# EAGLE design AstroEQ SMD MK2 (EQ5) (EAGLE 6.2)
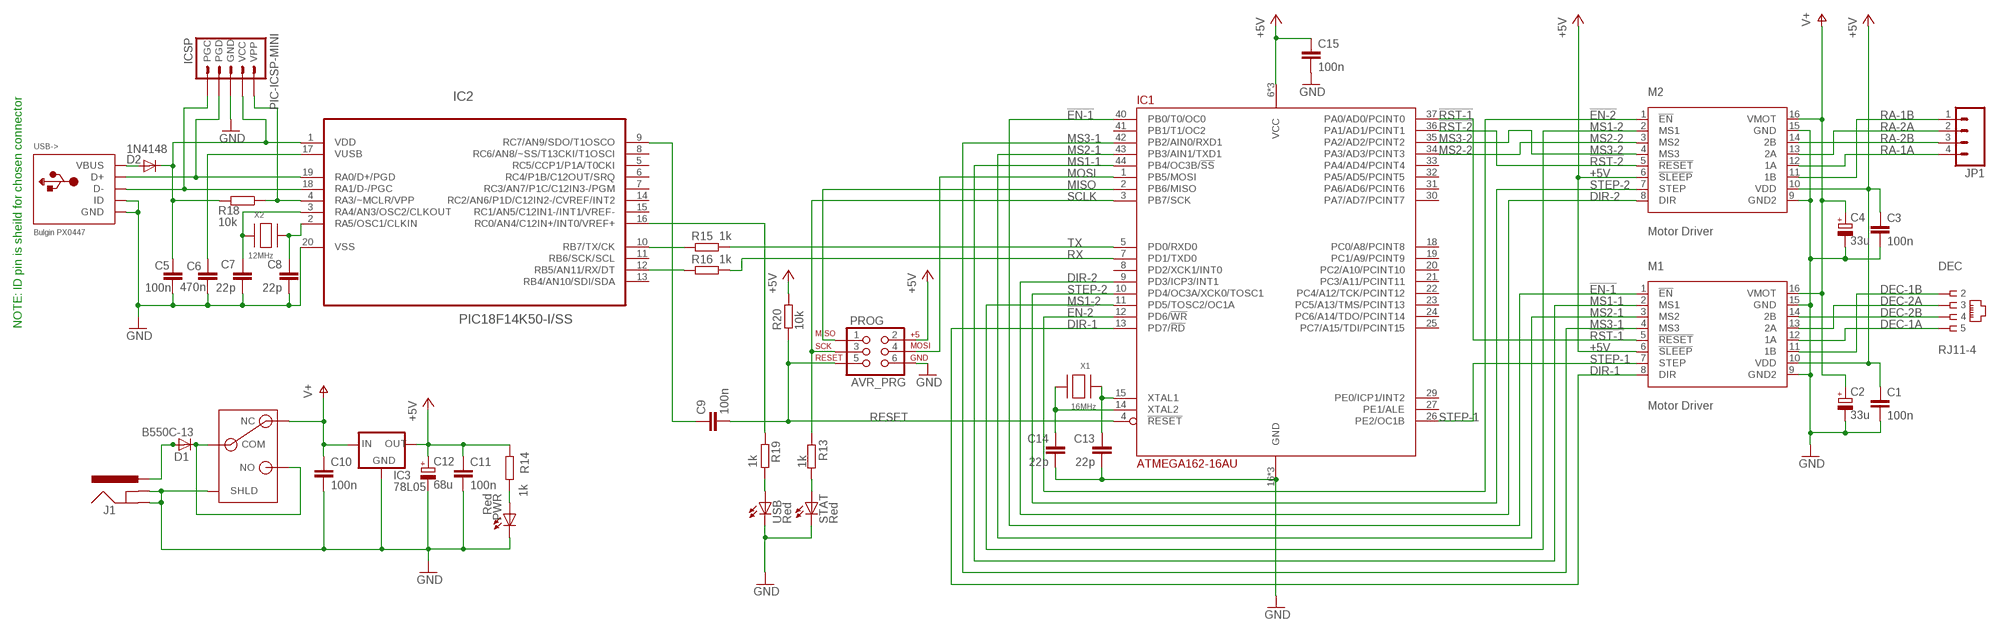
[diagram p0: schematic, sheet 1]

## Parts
C1  100n  C-EUC0603  [C0603]
C2  33u  CPOL-EUC/6032-28R  [C/6032-28R]
C3  100n  C-EUC0603  [C0603]
C4  33u  CPOL-EUC/6032-28R  [C/6032-28R]
C5  100n  C-EUC0603  [C0603]
C6  470n  C-EUC0603  [C0603]
C7  22p  C-EUC0603  [C0603]
C8  22p  C-EUC0603  [C0603]
C9  100n  C-EUC0603  [C0603]
C10  100n  C-EUC0603  [C0603]
C11  100n  C-EUC0603  [C0603]
C12  68u  CPOL-EUC/6032-28R  [C/6032-28R]
C13  22p  C-EUC0603  [C0603]
C14  22p  C-EUC0603  [C0603]
C15  100n  C-EUC0603  [C0603]
D1  B550C-13  DIODE-SMC  [SMC]
D2  1N4148  DIODESOD  [SOD-323]
DEC  RJ11-4  [RJ11-NO_SHIELD-4]
IC1  ATMEGA162-16AU  [TQFP44]
IC2  PIC18F14K50-I/SS  [SS20]
IC3  78L05  78LXXSOT-23  [SOT23]
ICSP  PIC-ICSP-MINI  [PIC-ICSP-MINI]
J1  POWER_JACKPANEL  [POWER_JACK_PANEL]
JP1  M04POLAR  [MOLEX-1X4]
M1  Motor Driver  A4983CARRIER  [DIP16-W]
M2  Motor Driver  A4983CARRIER  [DIP16-W]
PROG  AVR_PRG  AVR_SPI_PRG_6PTH  [2X3]
PWR  Red  LED3MM  [LED3MM]
R13  1k  R-EU_R0603  [R0603]
R14  1k  R-EU_R0603  [R0603]
R15  1k  R-EU_R0603  [R0603]
R16  1k  R-EU_R0603  [R0603]
R18  10k  R-EU_R0603  [R0603]
R19  1k  R-EU_R0603  [R0603]
R20  10k  R-EU_R0603  [R0603]
STAT  Red  LED3MM  [LED3MM]
SW1  SWITCH  [SPST]
USB  Red  LED3MM  [LED3MM]
USB->  Bulgin PX0447  USBBULGIN  [USB-MINIB-BULGIN]
X1  16MHz  XTALNX5032  [NX5032]
X2  12MHz  XTALNX5032  [NX5032]

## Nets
!EN-1: IC1.40(PB0/T0/OC0) M1.1(!EN)
!EN-2: IC1.12(PD6/!WR) M2.1(!EN)
!RST-1: IC1.37(PA0/AD0/PCINT0) M1.5(!RESET)
!RST-2: IC1.36(PA1/AD1/PCINT1) M2.5(!RESET)
+5V: C1.1 C3.1 C11.1 C12.+ C15.1 IC1.6(VCC) IC1.17(VCC) IC1.38(VCC) IC3.1(OUT) M1.6(!SLEEP) M1.10(VDD) M2.6(!SLEEP) M2.10(VDD) PROG.2 R14.1 R20.2
AVROSC1: C13.1 IC1.15(XTAL1) X1.P$1
AVROSC2: C14.1 IC1.14(XTAL2) X1.P$2
D+: IC2.19(RA0/D+/PGD) ICSP.4(PGD) USB->.3(D+)
D-: IC2.18(RA1/D-/PGC) ICSP.5(PGC) USB->.2(D-)
DEC-1A: DEC.5 M1.12(1A)
DEC-1B: DEC.2 M1.11(1B)
DEC-2A: DEC.3 M1.13(2A)
DEC-2B: DEC.4 M1.14(2B)
DIR-1: IC1.13(PD7/!RD) M1.8(DIR)
DIR-2: IC1.9(PD3/ICP3/INT1) M2.8(DIR)
DTR: C9.1 IC2.9(RC7/AN9/SDO/T1OSCO)
GND: C1.2 C2.- C3.2 C4.- C5.2 C6.1 C7.2 C8.2 C10.2 C11.2 C12.- C13.2 C14.2 C15.2 IC1.16(GND) IC1.28(GND) IC1.39(GND) IC2.20(VSS) IC3.3(GND) ICSP.3(GND) J1.SHUNT(GNDBREAK) J1.SLEEVE(GND) M1.9(GND2) M1.15(GND) M2.9(GND2) M2.15(GND) PROG.6 PWR.K(C) STAT.K(C) SW1.S1(SHLD) SW1.S2(SHLD) SW1.S3(SHLD) SW1.S4(SHLD) USB->.4(GND) USB->.5(ID) USB.K(C)
MCLR: IC2.4(RA3/~MCLR/VPP) ICSP.1(VPP) R18.1
MISO: IC1.2(PB6/MISO) PROG.1
MOSI: IC1.1(PB5/MOSI) PROG.4
MS1-1: IC1.44(PB4/OC3B/!SS) M1.2(MS1)
MS1-2: IC1.11(PD5/TOSC2/OC1A) M2.2(MS1)
MS2-1: IC1.43(PB3/AIN1/TXD1) M1.3(MS2)
MS2-2: IC1.34(PA3/AD3/PCINT3) M2.3(MS2)
MS3-1: IC1.42(PB2/AIN0/RXD1) M1.4(MS3)
MS3-2: IC1.35(PA2/AD2/PCINT2) M2.4(MS3)
PWRLED: PWR.A R14.2
RA-1A: JP1.4 M2.12(1A)
RA-1B: JP1.1 M2.11(1B)
RA-2A: JP1.2 M2.13(2A)
RA-2B: JP1.3 M2.14(2B)
RESET: C9.2 IC1.4(!RESET) PROG.5 R20.1
RX: IC1.7(PD1/TXD0) R16.1
RX(USB): IC2.12(RB5/AN11/RX/DT) R16.2
SCLK: IC1.3(PB7/SCK) PROG.3 R13.1
STATLED: R13.2 STAT.A
STEP-1: IC1.26(PE2/OC1B) M1.7(STEP)
STEP-2: IC1.10(PD4/OC3A/XCK0/TOSC1) M2.7(STEP)
SWITCH: D1.C SW1.COM SW1.NO
TX: IC1.5(PD0/RXD0) R15.1
TX(USB): IC2.10(RB7/TX/CK) R15.2
USBLED: R19.1 USB.A
USBOSC1: C8.1 IC2.2(RA5/OSC1/CLKIN) X2.P$2
USBOSC2: C7.1 IC2.3(RA4/AN3/OSC2/CLKOUT) X2.P$1
USBSTAT: IC2.16(RC0/AN4/C12IN+/INT0/VREF+) R19.2
V+: C2.+ C4.+ C10.1 IC3.2(IN) M1.16(VMOT) M2.16(VMOT) SW1.NC
VBUS: D2.2(A) USB->.1(VBUS)
VIN: D1.A J1.CENTRE(PWR)
VPIC: C5.1 D2.1(C) IC2.1(VDD) ICSP.2(VCC) R18.2
VUSB: C6.2 IC2.17(VUSB)
Unconnected: IC1.8(PD2/XCK1/INT0) IC1.18(PC0/A8/PCINT8) IC1.19(PC1/A9/PCINT9) IC1.20(PC2/A10/PCINT10) IC1.21(PC3/A11/PCINT11) IC1.22(PC4/A12/TCK/PCINT12) IC1.23(PC5/A13/TMS/PCINT13) IC1.24(PC6/A14/TDO/PCINT14) IC1.25(PC7/A15/TDI/PCINT15) IC1.27(PE1/ALE) IC1.29(PE0/ICP1/INT2) IC1.30(PA7/AD7/PCINT7) IC1.31(PA6/AD6/PCINT6) IC1.32(PA5/AD5/PCINT5) IC1.33(PA4/AD4/PCINT4) IC1.41(PB1/T1/OC2) IC2.5(RC5/CCP1/P1A/T0CKI) IC2.6(RC4/P1B/C12OUT/SRQ) IC2.7(RC3/AN7/P1C/C12IN3-/PGM) IC2.8(RC6/AN8/~SS/T13CKI/T1OSCI) IC2.11(RB6/SCK/SCL) IC2.13(RB4/AN10/SDI/SDA) IC2.14(RC2/AN6/P1D/C12IN2-/CVREF/INT2) IC2.15(RC1/AN5/C12IN1-/INT1/VREF-)

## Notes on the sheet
- NOTE: ID pin is sheild for chosen connector

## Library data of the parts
C1 C3 C5 C9-C11 C15 = resistor:C-EU: CAPACITOR, European symbol; MF: MULTICOMP; MPN: T0603F104ZCT; OC_FARNELL: 9406204
C2 C4 = resistor:CPOL-EU: POLARIZED CAPACITOR, European symbol; MF: KEMET; MPN: T491C336K025AT; OC_FARNELL: 1793896
C6 = rcl:C-EU: CAPACITOR, European symbol; MF: MURATA; MPN: GRM188R61C474KA93D; OC_FARNELL: 1828894
C7 C8 C13 C14 = rcl:C-EU: CAPACITOR, European symbol; MF: MULTICOMP; MPN: U0603C220JCT; OC_FARNELL: 9406107
C12 = resistor:CPOL-EU: POLARIZED CAPACITOR, European symbol; MF: AVX; MPN: TPSC686K016R0125; OC_FARNELL: 1658976
D1 = diode:DIODE-: DIODE; MF: DIODES INC.; MPN: B550C-13-F; OC_FARNELL: 1858608
D2 = SparkFun:DIODE: Diode; MF: VISHAY SEMICONDUCTOR; MPN: 1N4148WS-V-GS08; OC_FARNELL: 1617737
DEC = con-tycoelectronics:RJ11-4; MF: MOLEX; MPN: 95503-2641; OC_FARNELL: 1572017
IC1 = atmel:ATMEGA162: 8-bit RISC MICROCONTROLLER 16K Bytes internal flash program memory 1K Bytes internal SRAM Upto 64K Bytes optional external memory space 512 Bytes EEPROM Two 8-bit timers Two 16-bit timers Dual programmable serial USARTs Master/Slave serial SPI interface Source: ATMEGA162_DIP40.lbr; MF: ATMEL; MPN: ATMEGA162-16AU; OC_FARNELL: 9171150
IC2 = microchip:PIC18F14K50: USB Flash Microcontrollers; MF: MICROCHIP; MPN: PIC18F14K50-I/SS; OC_FARNELL: 1648504; PACKAGE: SSOP20; SUPPLIER: Microchip
IC3 = v-reg:78LXX: VOLTAGE REGULATOR; MF: TAIWAN SEMICONDUCTOR; MPN: TS78L05CX RF; OC_FARNELL: 1476698
ICSP = SparkFun:PIC-ICSP-MINI: PIC-ICSP-Mini Miniature 5-pin connection for temporary programming of PICs. Use this device in your design to save space. Program the PIC with this adapter Spark Fun Electronics SKU : BOB-00194; MF: HARWIN; MPN: M52-5000545; OC_FARNELL: 1099543
J1 = SparkFun:POWER_JACK: Power Jack This is the standard 5.5mm barrel jack for power. The PTH is the most common, proven, reliable, footprint. All others are experimental. The Slot footprint only works if the mill layer is transmitted to the PCB fab house so be warned. Spark Fun Electronics SKU : PRT-00119. Mating wall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; MF: SWITCHCRAFT; MPN: PCL712AS; OC_FARNELL: 1871167
JP1 = SparkFun:M04: Header 4 Standard 4-pin 0.1" header. Use with straight break away headers (SKU : PRT-00116), right angle break away headers (PRT-00553), swiss pins (PRT-00743), machine pins (PRT-00117), and female headers (PRT-00115). Molex polarized connector foot print use with SKU : PRT-08231 with associated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; MF: MULTICOMP; MPN: MC34645; OC_FARNELL: 1675775
M1 M2 = A4983Carrier:A4983CARRIER; OC_FARNELL: unknown
PROG = SparkFun:AVR_SPI_PRG_6: AVR ISP 6 Pin This is the reduced ISP connector for AVR programming. Common on Arduino. This footprint will take up less PCB space and can be used with a 10-pin to 6-pin adapter such as SKU: BOB-08508; MF: TE CONNECTIVITY / AMP; MPN: 826632-3; OC_FARNELL: 3418492
PWR STAT USB = led:LED: LED; MF: KINGBRIGHT; MPN: L-424HDT; OC_FARNELL: 1142499
R13 R14 R19 = rcl:R-EU_: RESISTOR, European symbol; MF: PANASONIC; MPN: ERJ3GEYJ102V; OC_FARNELL: 2059601
R15 R16 = SmartPrj:R-EU_: RESISTOR, European symbol; MF: PANASONIC; MPN: ERJ3GEYJ102V; OC_FARNELL: 2059601
R18 R20 = rcl:R-EU_: RESISTOR, European symbol; MF: PANASONIC; MPN: ERJ3GEYJ103V; OC_FARNELL: 2059627
SW1 = con-tycoelectronics:SWITCH; MF: TE CONNECTIVITY; MPN: AE101J1V3B004; OC_FARNELL: 1813654
USB-> = adafruit:USB: USB Connectors USBMINIB - Surface Mount Female Mini-B USB Connector 4UConnector: 06564 By microbuilder.eu Thru-hole RA Female Mini-B USB Connector 4UConnector: 18732 By ladyada.net; MF: BULGIN; MPN: PX0447; OC_FARNELL: 1229687
X1 = adafruit:XTAL: Low cost SMT crystals, no capacitors included; MF: TXC; MPN: 7A-16.000MAAJ-T; OC_FARNELL: 1841946
X2 = adafruit:XTAL: Low cost SMT crystals, no capacitors included; MF: TXC; MPN: 7A-12.000MAAJ-T; OC_FARNELL: 1841940

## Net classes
1 power: width 0.61 mm, drill 0.711 mm, clearance 0.203 mm
2 gnd: width 0.305 mm, drill 0.711 mm, clearance 0.203 mm
3 usbvcc: width 0.508 mm, drill 0.711 mm, clearance 0.203 mm

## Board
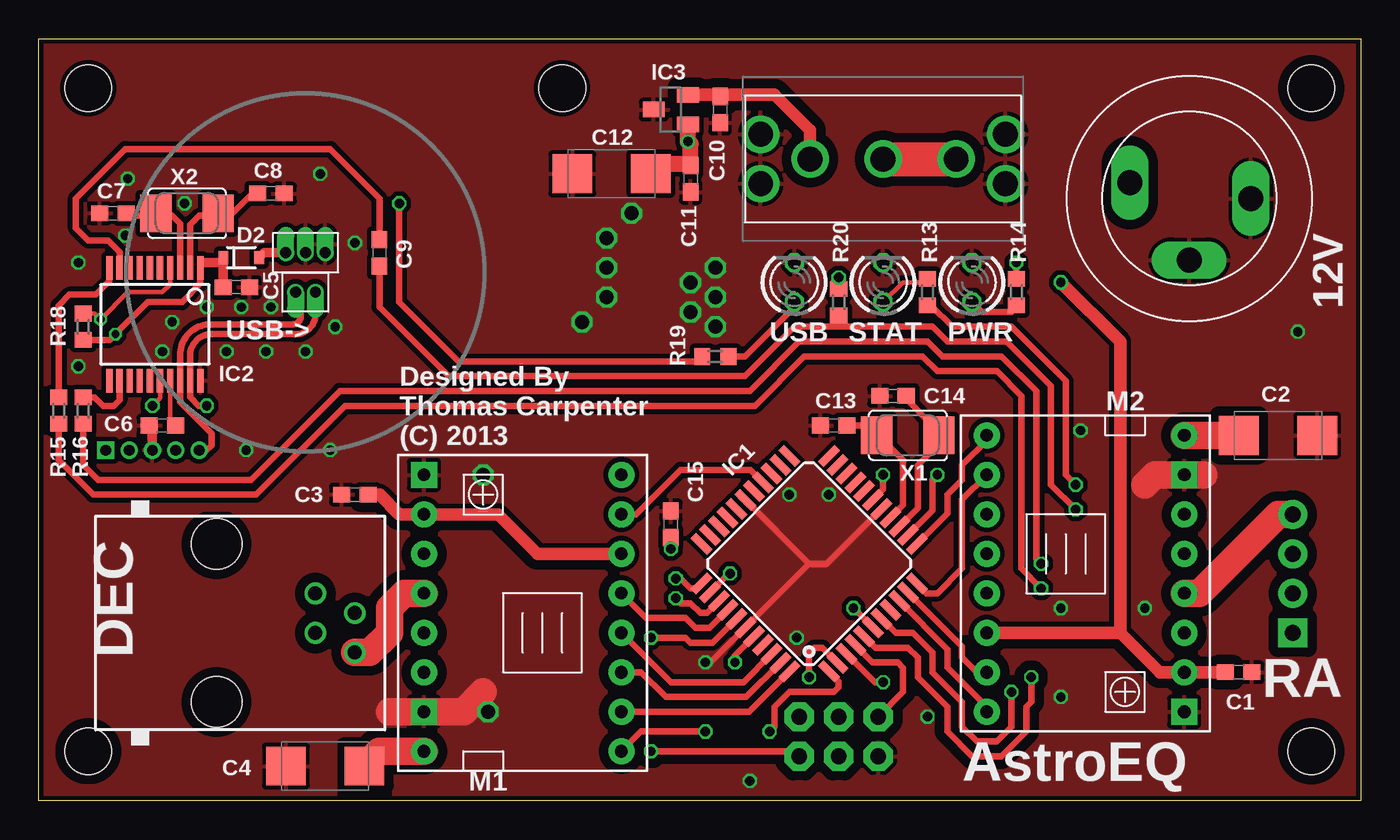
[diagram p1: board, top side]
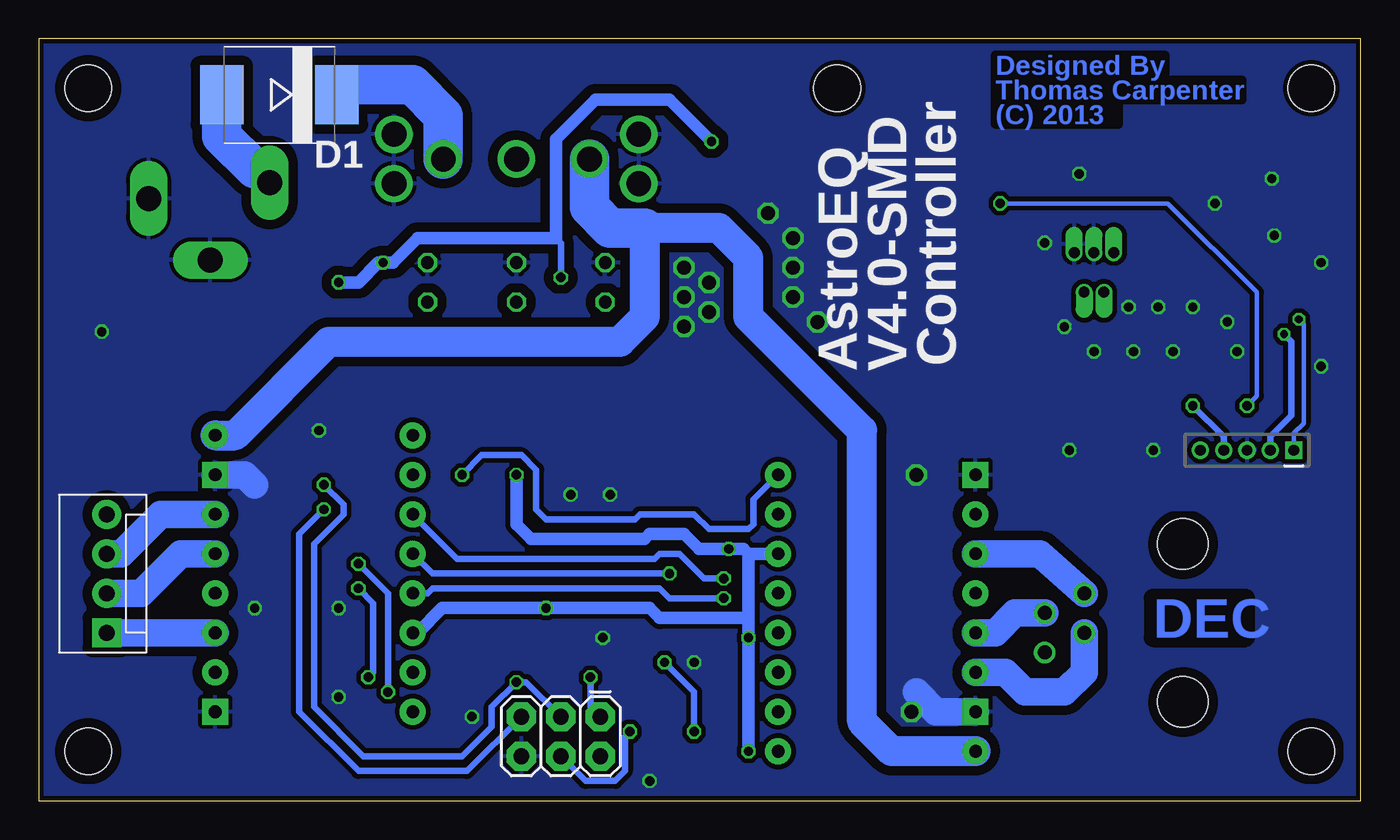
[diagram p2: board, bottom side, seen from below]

Size 85 x 49 mm. Coordinates in mm from the lower left corner, seen from the top.
Outline: 0,0 0,49 85,49 85,0 0,0
Copper layers (1*16): Top 0.035mm / dielectric 1.5mm / Bottom 0.035mm
Design rules: minimum track width 6mil, minimum drill 12mil, track to track 6mil, track to pad 6mil, pad to pad 6mil, via to via 6mil, smd to smd 0mil, copper to edge 10mil, drill to drill 10mil, minimum pad ring 8mil, minimum via ring 6mil, stop-mask expansion 2mil, vias tented up to drill 1mm, thermal gap 10mil
Holes 3 mm at 81.83,3.17 33.66,45.83 3.17,45.83 81.83,45.83 3.17,3.17
tKeepout: area 78.3,7.4 to 83.3,12.4; area 78.3,53.6 to 83.3,58.6; area 48.3,7.4 to 53.3,12.4; area 8.3,7.4 to 13.3,12.4; area 48.3,53.6 to 53.3,58.6; area 8.3,53.6 to 13.3,58.6
bKeepout: area 78.3,7.4 to 83.3,12.4; area 78.3,53.6 to 83.3,58.6; area 48.3,7.4 to 53.3,12.4; area 8.3,7.4 to 13.3,12.4; area 48.3,53.6 to 53.3,58.6; area 8.3,53.6 to 13.3,58.6

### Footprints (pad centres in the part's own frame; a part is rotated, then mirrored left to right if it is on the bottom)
C0603 = smd 1.1 x 1: 1 -0.85,0; 2 0.85,0
C/6032-28R = smd 2.55 x 2.5: + 2.525,0; - -2.525,0
SMC = smd 2.8 x 3.8: A 3.7,0; C -3.7,0
SOD-323 = smd 0.63 x 0.83: 1 -1.15,0; 2 1.15,0
RJ11-NO_SHIELD-4 = drill 0.9 pad 1.4: 2 -1.905,6.35; 3 -0.635,8.89; 4 0.635,6.35; 5 1.905,8.89 | hole 3.251: -5.08,0; 5.08,0
TQFP44 = smd 1.5 x 0.5: 1 -5.8,4; 2 -5.8,3.2; 3 -5.8,2.4; 4 -5.8,1.6; 5 -5.8,0.8; 6 -5.8,0; 7 -5.8,-0.8; 8 -5.8,-1.6; 9 -5.8,-2.4; 10 -5.8,-3.2; 11 -5.8,-4; 23 5.8,-4; 24 5.8,-3.2; 25 5.8,-2.4; 26 5.8,-1.6; 27 5.8,-0.8; 28 5.8,0; 29 5.8,0.8; 30 5.8,1.6; 31 5.8,2.4; 32 5.8,3.2; 33 5.8,4 | smd 0.5 x 1.5: 12 -4,-5.8; 13 -3.2,-5.8; 14 -2.4,-5.8; 15 -1.6,-5.8; 16 -0.8,-5.8; 17 0,-5.8; 18 0.8,-5.8; 19 1.6,-5.8; 20 2.4,-5.8; 21 3.2,-5.8; 22 4,-5.8; 34 4,5.8; 35 3.2,5.8; 36 2.4,5.8; 37 1.6,5.8; 38 0.8,5.8; 39 0,5.8; 40 -0.8,5.8; 41 -1.6,5.8; 42 -2.4,5.8; 43 -3.2,5.8; 44 -4,5.8
SS20 = smd 0.4 x 1.5: 1 -2.925,-3.625; 2 -2.275,-3.625; 3 -1.625,-3.625; 4 -0.975,-3.625; 5 -0.325,-3.625; 6 0.325,-3.625; 7 0.975,-3.625; 8 1.625,-3.625; 9 2.275,-3.625; 10 2.925,-3.625; 11 2.925,3.625; 12 2.275,3.625; 13 1.625,3.625; 14 0.975,3.625; 15 0.325,3.625; 16 -0.325,3.625; 17 -0.975,3.625; 18 -1.625,3.625; 19 -2.275,3.625; 20 -2.925,3.625
SOT23 = smd 1 x 1.4: 1 -0.95,-1.1; 2 0.95,-1.1; 3 0,1.1
PIC-ICSP-MINI = drill 0.7 square: 1 -3,0 | drill 0.7: 2 -1.5,0; 3 0,0; 4 1.5,0; 5 3,0
POWER_JACK_PANEL = drill 1.6 long: CENTRE 3.81,-1.016; SHUNT -3.962,0; SLEEVE 0,3.962
MOLEX-1X4 = drill 1.016 pad 1.88 square: 1 0,0 | drill 1.016 pad 1.88: 2 2.54,0; 3 5.08,0; 4 7.62,0
DIP16-W = drill 0.813 pad 1.676: 1 -8.89,-6.35; 2 -6.35,-6.35; 3 -3.81,-6.35; 4 -1.27,-6.35; 5 1.27,-6.35; 6 3.81,-6.35; 7 6.35,-6.35; 8 8.89,-6.35; 10 6.35,6.35; 11 3.81,6.35; 12 1.27,6.35; 13 -1.27,6.35; 14 -3.81,6.35; 16 -8.89,6.35 | drill 0.813 pad 1.676 square: 9 8.89,6.35; 15 -6.35,6.35
2X3 = drill 1.016 pad 1.88 octagon: 1 0,0; 2 0,2.54; 3 2.54,0; 4 2.54,2.54; 5 5.08,0; 6 5.08,2.54
LED3MM = drill 0.813 octagon: A -1.27,0; K 1.27,0
R0603 = smd 1 x 1.1: 1 -0.85,0; 2 0.85,0
SPST = drill 1.6: COM 0,0; NC -4.699,0; NO 4.699,0; S1 7.874,1.587; S2 7.874,-1.587; S3 -7.874,1.587; S4 -7.874,-1.587
USB-MINIB-BULGIN = drill 0.7 pad 1.016 offset: 1 -1.27,1.27; 2 -0.635,-1.27; 3 0.635,-1.27; 4 0,1.27; 5 1.27,1.27
NX5032 = smd 2 x 2.4: P$1 2,0; P$2 -2,0

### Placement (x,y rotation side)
C1  77.15,8.26 0 top
C2  79.69,23.5 180 top
C3  20.32,19.68 180 top
C4  18.41,2.22 0 top
C5  12.7,33.02 0 top
C6  7.94,24.13 0 top
C7  4.76,37.78 180 top
C8  14.92,39.05 0 top
C9  21.91,35.24 270 top
C10  43.81,44.45 270 top
C11  41.91,40.01 270 top
C12  36.83,40.32 0 top
C13  51.12,24.13 180 top
C14  54.93,26.04 180 top
C15  40.64,17.78 90 top
D1  69.53,45.4 180 bottom
D2  13.02,34.92 0 top
DEC  11.43,11.43 270 top
IC1  49.53,15.24 135 top
IC2  7.46,30.64 180 top
IC3  40.64,44.45 90 top
ICSP  7.3,22.54 180 bottom
J1  73.98,38.73 180 top
JP1  80.64,10.79 90 bottom
M1  31.11,12.06 90 top
M2  67.31,14.61 270 top
PROG  48.9,5.4 180 bottom
PWR  60.01,33.34 90 top
R13  57.15,32.7 90 top
R14  62.87,32.7 270 top
R15  1.27,25.08 90 top
R16  2.86,25.08 90 top
R18  2.86,30.48 270 top
R19  43.5,28.57 180 top
R20  51.44,32.07 90 top
STAT  54.29,33.34 90 top
SW1  54.29,41.27 0 top
USB  48.58,33.34 90 top
USB->  17.14,33.97 0 top
X1  55.88,23.5 180 top
X2  9.53,37.78 180 top

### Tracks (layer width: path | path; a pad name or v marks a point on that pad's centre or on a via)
!EN-1  (via drill 0.6)
  Top 0.406: IC1.40 44.77,9.35 v44.77,8.89 | M1.1 38.73,4.45 v42.86,4.45
  Bottom 0.406: v44.77,8.89 42.86,6.99 v42.86,4.45
!EN-2
  Top 0.406: IC1.12 58.42,18.47 58.42,19.68 59.37,20.64 59.37,21.59 60.96,23.18 M2.1
!RST-1
  Top 0.406: IC1.37 43.14,11.11 42.23,11.11 41.59,11.75 39.05,11.75 M1.5
!RST-2  (via drill 0.6)
  Top 0.406: IC1.36 42.96,12.06 42.55,12.06 41.91,12.7 41.27,12.7 v40.96,13.02
  Bottom 0.406: v40.96,13.02 44.45,13.02 45.09,13.65 59.69,13.65 60.01,13.34 M2.5
+5V  (via drill 0.6)
  Top 0.406: IC1.38 43.32,10.16 41.91,10.16 41.59,10.48 v39.37,10.48 | IC1.6 v52.39,12.38 | PROG.2 48.58,3.17 v39.37,3.17 | IC1.17 54.29,20 v54.29,20.95 | R20.2 v51.44,33.66 | R14.1 v62.87,34.61
  Top 0.813: C3.1 21.91,19.68 23.18,18.41 M1.10 29.53,18.41 32.07,15.88 M1.6 | 69.53,10.79 72.07,8.26 M2.10 C1.1 | 69.53,10.79 M2.6 | 69.53,10.79 69.53,29.53 v65.72,33.34 | C15.1 v40.64,16.19
  Top 1.016: IC3.1 v41.74,42.4 41.91,42.23 41.91,40.96 | C12.+ 39.66,40.32 40.3,40.96 41.91,40.96 | C11.1 41.91,40.96
  Bottom 0.406: 51.75,36.2 51.44,35.88 v51.44,33.66
  Bottom 0.813: 39.37,11.75 45.09,11.75 45.72,12.38 v52.39,12.38 59.05,12.38 60.64,10.79 M2.6 | v39.37,3.17 v39.37,10.48 39.37,11.75 | M1.6 39.37,15.88 | 39.37,15.88 39.37,11.75 | v54.29,20.95 54.29,17.78 53.34,16.83 46.04,16.83 45.72,17.14 43.5,17.14 42.55,16.19 v40.64,16.19 39.69,16.19 39.37,15.88 | v65.72,33.34 64.45,33.34 63.18,34.61 v62.87,34.61 62.23,34.61 60.64,36.2 51.75,36.2 51.75,42.55 49.21,45.09 44.45,45.09 41.91,42.55 v41.74,42.4
AVROSC1
  Top 0.406: IC1.15 55.56,19.01 55.56,21.91 53.98,23.5 X1.P$1 53.24,24.13 C13.1
AVROSC2
  Top 0.406: IC1.14 56.52,18.83 56.52,21.59 57.78,22.86 X1.P$2 57.68,23.69 57.68,23.91 55.78,25.82 C14.1
D+  (via drill 0.6)
  Top 0.406: USB->.3 17.78,31.27 arc-90 16.51,30 10.95,30 arc90 9.74,28.47 IC2.19 9.74,25.95 10.29,25.4 v10.79,25.4
  Bottom 0.406: ICSP.4 8.8,23.41 v10.79,25.4
D-
  Top 0.406: USB->.2 arc-90 16.83,32.38 16.83,31.11 arc-90 16.35,30.64 10.95,30.64 arc90 9.09,28.61 IC2.18 9.09,25.65 11.11,23.62 11.11,22.86 10.79,22.54 ICSP.5
DEC-1A
  Top 1.778: DEC.5 21.27,9.53 22.54,10.79 22.54,12.38 23.5,13.34 M1.12
DEC-1B
  Bottom 1.778: M1.11 20.64,15.88 DEC.2
DEC-2A
  Bottom 1.778: DEC.3 22.23,12.06 23.5,10.79 M1.13
DEC-2B
  Bottom 1.778: M1.14 22.86,8.26 21.59,6.99 19.05,6.99 17.78,8.26 DEC.4
DIR-1  (via drill 0.6)
  Top 0.406: IC1.13 57.47,18.65 57.47,20.64 v57.78,20.95
  Bottom 0.406: M1.8 39.05,19.37 39.05,17.78 39.37,17.46 41.91,17.46 42.86,18.41 46.35,18.41 46.67,18.1 52.39,18.1 53.02,18.73 53.02,21.27 53.98,22.23 56.52,22.23 v57.78,20.95
DIR-2
  Top 0.406: IC1.9 58.42,9.74 58.42,8.57 60.96,6.03 M2.8
DTR
  Top 0.406: IC2.9 5.19,35.3 4.45,36.04 3.17,36.04 2.38,36.83 2.38,38.73 5.56,41.91 18.73,41.91 21.91,38.73 C9.1
GND  (via drill 0.6, 0.9)
  Top 0.406: 43.18,8.89 IC1.39 49.53,15.24 | IC1.16 50.66,15.24 49.53,15.24 | IC1.28 49.53,15.24 | 49.53,15.24
  Top 0.61: C6.1 7.3,23.91 ICSP.3
  Top 1.778: 28.57,6.99 27.3,5.71 M1.15 22.54,5.71 | 71.12,20.32 71.75,20.95 M2.15 74.93,20.95
  Bottom 1.778: M1.15 27.3,5.71 28.57,6.99 | M2.15 71.75,20.95 71.12,20.32
  other vias: 71.12,12.38 57.15,5.4 42.86,8.89 48.26,19.68 20.32,35.88 80.96,30.16 18.1,40.32 65.72,12.38 50.8,19.68 18.73,22.54 7.94,28.89 66.99,23.81 14.61,28.89 48.74,10.48 5.71,40.01 19.05,30.48 17.14,28.89 13.02,31.75 8.57,30.8 14.92,31.75 10.79,31.75 9.37,38.42 12.06,28.89 5.56,36.35 13.34,22.54 2.54,34.61 2.54,27.94 45.72,1.27 65.72,6.67 43.5,34.29 41.91,33.34 41.91,31.43 36.51,34.29 36.51,32.38 34.92,30.8 28.57,20.95 28.89,5.71 36.51,36.2 38.1,37.78 43.5,32.38 43.5,30.48
  pour Top (isolate 0.61, rank 3): 30.16,50.16 85.79,50.16 85.79,-0.95 -2.54,-0.95 -2.54,19.68 30.16,19.68
  pour Bottom (isolate 0.61): 30.16,49.85 85.79,49.85 85.79,-1.27 -2.54,-1.27 -2.54,19.68 15.56,19.68 16.19,20.32 30.16,20.32
  pour Top (isolate 0.305): -2.54,50.8 -2.54,-1.59 0.95,-1.59 0.95,18.73 14.61,18.73 15.56,19.68 21.91,19.68 23.18,18.41 29.53,18.41 32.07,15.88 37.47,15.88 37.47,3.17 44.77,3.17 46.99,5.4 53.66,5.4 59.05,10.79 65.41,10.79 67.94,8.26 73.66,8.26 73.66,8.89 73.34,8.89 70.48,11.75 70.48,32.7 65.09,37.78 43.81,37.78 43.81,43.81 40.32,43.81 40.32,48.26 83.5,48.26 84.14,48.26 84.14,-2.22 87.31,-2.22 87.31,48.26 87.31,50.8
  pour Bottom (isolate 0.305): -2.54,50.8 -2.54,-2.22 0.95,-2.22 0.95,18.73 14.61,18.73 16.19,20.32 30.16,20.32 30.16,38.42 36.51,44.77 36.51,48.26 84.14,48.26 84.14,-2.22 87.31,-2.22 87.31,50.8
  pour Bottom (isolate 0.305): 35.24,23.5 35.24,0.95 0.95,0.95 0.95,-2.22 84.14,-2.22 84.14,0.95 70.48,0.95 70.48,21.91 63.5,21.91 63.5,25.4 61.28,27.62 39.37,27.62
  pour Top (isolate 0.305, rank 2): 0.95,-2.22 0.95,0.95 13.34,0.95 13.34,4.13 19.05,4.13 19.05,0.32 22.86,0.32 22.86,0.64 45.09,0.64 45.09,1.91 46.67,1.91 46.67,0.64 85.72,0.64 85.72,-2.22
MCLR  (via drill 0.5)
  Top 0.305: IC2.4 8.44,33.2 7.94,32.7 5.71,32.7 v3.97,30.96 3.6,31.33 R18.1
  Bottom 0.305: v3.97,30.96 3.67,30.66 3.67,24.27 4.3,23.64 ICSP.1
MISO  (via drill 0.6)
  Top 0.406: IC1.2 50.4,9.84 49.85,9.84 49.53,9.53 v49.53,7.94
  Bottom 0.406: PROG.1 49.53,6.03 v49.53,7.94
MOSI  (via drill 0.6)
  Top 0.406: IC1.1 51.44,7.68 51.44,7.3 51.12,6.99 48.26,6.99 47.31,6.03 47.31,4.76 v46.99,4.45
  Bottom 0.406: v46.99,4.45 47.31,4.13 47.31,1.91 47.94,1.27 49.85,1.27 PROG.4
MS1-1
  Top 0.406: IC1.44 45.66,5.71 M1.2
MS1-2
  Top 0.406: IC1.11 57.09,13.34 57.78,13.34 59.37,14.92 59.37,19.37 M2.2
MS2-1
  Top 0.406: M1.3 38.73,8.26 40.32,6.67 45.48,6.67 IC1.43
MS2-2  (via drill 0.6)
  Top 0.406: IC1.34 42.29,13.65 41.91,13.65 41.27,14.29 v40.96,14.29
  Bottom 0.406: M2.3 58.1,15.56 45.4,15.56 45.09,15.88 43.81,15.88 42.23,14.29 v40.96,14.29
MS3-1
  Top 0.406: M1.4 40.64,7.62 45.3,7.62 IC1.42
MS3-2  (via drill 0.6)
  Top 0.406: IC1.35 44.37,14.61 v44.45,14.61
  Bottom 0.406: v44.45,14.61 59.69,14.61 M2.4
PWRLED
  Top 0.406: PWR.A 60.64,31.43 62.55,31.43 62.87,31.75 R14.2
RA-1A
  Top 1.778: M2.12 74.61,13.34 79.69,18.41 JP1.4
RA-1B
  Bottom 1.778: JP1.1 M2.11
RA-2A
  Bottom 1.778: M2.13 75.88,15.88 78.42,13.34 JP1.2
RA-2B
  Bottom 1.778: M2.14 77.15,18.41 79.69,15.88 JP1.3
RESET  (via drill 0.6)
  Top 0.406: IC1.4 53.62,8.89 55.24,8.89 55.56,8.53 55.56,6.99 PROG.5 | v66.67,18.73 65.09,20.32 65.09,26.67 62.23,29.53 58.42,29.53 57.47,30.48 51.44,30.48 | 51.44,30.48 48.58,30.48 45.4,27.3 26.35,27.3 21.91,31.75 C9.2 | R20.1 51.44,30.48
  Bottom 0.406: v66.67,18.73 68.26,17.14 68.26,5.71 64.45,1.91 57.47,1.91 PROG.5
RX  (via drill 0.6)
  Top 0.406: R16.1 2.86,21.59 3.81,20.64 13.65,20.64 19.37,26.35 45.72,26.35 48.9,29.53 57.15,29.53 58.1,28.57 61.91,28.57 64.14,26.35 64.14,15.56 v64.45,15.24 | IC1.7 55.11,10.79 56.2,10.79 57.47,9.53 57.47,8.26 59.37,6.35 59.37,4.76 60.33,3.81 61.59,3.81 62.55,4.76 v62.55,6.99
  Bottom 0.406: v62.55,6.99 62.55,13.34 v64.45,15.24
RX(USB)
  Top 0.406: IC2.12 5.19,25.77 4.82,25.4 4.13,25.4 3.6,25.93 R16.2
SCLK  (via drill 0.6)
  Top 0.406: IC1.3 53.76,7.62 v54.29,7.62 | v66.67,20.32 66.04,20.95 66.04,26.99 62.55,30.48 58.74,30.48 57.37,31.85 R13.1
  Bottom 0.406: PROG.3 53.66,7.62 v54.29,7.62 55.88,6.03 55.88,4.76 57.78,2.86 64.14,2.86 67.31,6.03 67.31,16.51 65.41,18.41 65.41,19.05 v66.67,20.32
STATLED
  Top 0.305: R13.2 57.15,33.34 55.56,33.34 STAT.A
STEP-1
  Top 0.406: M1.7 38.42,18.41 41.27,21.27 45.76,21.27 IC1.26
STEP-2
  Top 0.406: IC1.10 59.37,9.92 59.37,9.21 60.33,8.26 M2.7
SWITCH
  Top 2.184: SW1.COM SW1.NO
  Bottom 2.184: D1.C 65.2,46.04 65.09,46.04
  Bottom 2.54: 65.09,46.04 60.96,46.04 58.99,44.07 SW1.NO
TX  (via drill 0.6)
  Top 0.406: R15.1 1.27,21.91 3.49,19.68 13.97,19.68 19.68,25.4 46.04,25.4 49.21,28.57 56.83,28.57 57.78,27.62 61.59,27.62 63.18,26.04 63.18,14.92 v64.45,13.65 | IC1.5 53.8,9.84 55.88,9.84 56.52,9.21 56.52,7.94 58.42,6.03 58.42,4.45 60.01,2.86 61.91,2.86 63.5,4.45 63.5,6.03 63.82,6.35 v63.82,7.94
  Bottom 0.406: v63.82,7.94 63.5,8.26 63.5,12.7 v64.45,13.65
TX(USB)
  Top 0.406: IC2.10 4.54,33.43 3.65,32.54 1.96,32.54 1.27,31.85 R15.2
USBLED
  Top 0.406: R19.1 45.4,28.57 48.58,31.75 USB.A
USBOSC1
  Top 0.406: IC2.2 9.74,37.04 10.32,37.62 11.53,37.62 | 11.53,37.62 12.3,37.62 13.73,39.05 C8.1 | X2.P$2 11.53,37.62
USBOSC2
  Top 0.406: IC2.3 9.09,37.11 8.57,37.62 7.53,37.62 | 7.53,37.62 5.77,37.62 C7.1 | X2.P$1 7.53,37.62
USBSTAT  (via drill 0.6)
  Top 0.305: IC2.16 7.79,25.88 v7.3,25.4
  Top 0.406: v23.18,38.42 23.18,32.07 26.99,28.26 42.33,28.26 R19.2
  Bottom 0.305: v7.3,25.4 6.67,26.04 6.67,32.7 12.38,38.42 v23.18,38.42
V+
  Top 0.813: SW1.NC 49.59,43.12 47.31,45.4 43.81,45.4 | 43.81,45.4 IC3.2 | C10.1 43.81,45.4
  Top 1.778: C4.+ 21.89,3.17 M1.16 | C2.+ M2.16
  Bottom 1.93: M1.16 30.16,3.17 32.07,5.08 32.07,23.81 39.37,31.11 39.37,34.92 41.27,36.83 46.04,36.83 46.04,31.11 47.62,29.53 66.36,29.53 72.39,23.5 M2.16
  Bottom 2.54: 46.04,36.83 48.26,36.83 49.59,38.16 SW1.NC
VBUS
  Top 0.61: USB->.1 14.48,35.24 D2.2
VIN
  Bottom 2.184: 71.12,40.64 71.06,40.64 J1.CENTRE
  Bottom 2.54: D1.A 73.23,42.75 71.12,40.64
VPIC  (via drill 0.5)
  Top 0.305: IC2.1 10.39,34.77 10.55,34.61
  Top 0.406: IC2.1 10.39,33.25 9.21,32.07 6.99,32.07 v4.92,30 4.55,29.63 R18.2
  Top 0.61: 10.55,34.61 11.75,34.61 11.87,34.73 D2.1 11.85,34.61 C5.1
  Bottom 0.406: v4.92,30 4.45,29.53 4.45,24.77 5.8,23.41 ICSP.2
VUSB
  Top 0.305: IC2.17 8.44,24.48 C6.2

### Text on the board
Bottom: Designed By | Thomas Carpenter | (C) 2013 | DEC
tNames: 12V | Designed By | Thomas Carpenter | (C) 2013 | RA | AstroEQ
bNames: Controller | V4.0-SMD | AstroEQ
Reference: This board design is for AstroEQ boards which fit inside the enclosure on an EQ5 Mount. | The board uses some very tricky surface mount components and is not recommended for DIY. | It is a 2 Layer board designed to be sent for manufacture. The AstroEQ-SMD-Gerber.zip file contains the required gerber files. | I use iteadstudio.com 10cm x 5cm prototype service, selecting 1.2mm thick, HASL, 100% electrical check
